FUNCTION "PALLET IMP.LAT. TRANSITO" : VOID
TITLE =
VERSION : 0.1
//KNOW_HOW_PROTECT

VAR_TEMP
  Error_block_move : INT ;
END_VAR
BEGIN
NETWORK
TITLE =Spostamento dati per pallet in transito tra impil. e ribaltat.
//- "Container Flag"
//- "Id TAG"
//- "FlagRibaltamento"
//- "Container_Id"
//- "Date LCB"
//- "Part Number"
//- "Quantity"
//- "Line Id"
//- "CIM"
//- "Colata Id"
//- "Material Of Test Flag"
//- "Lotto Id"
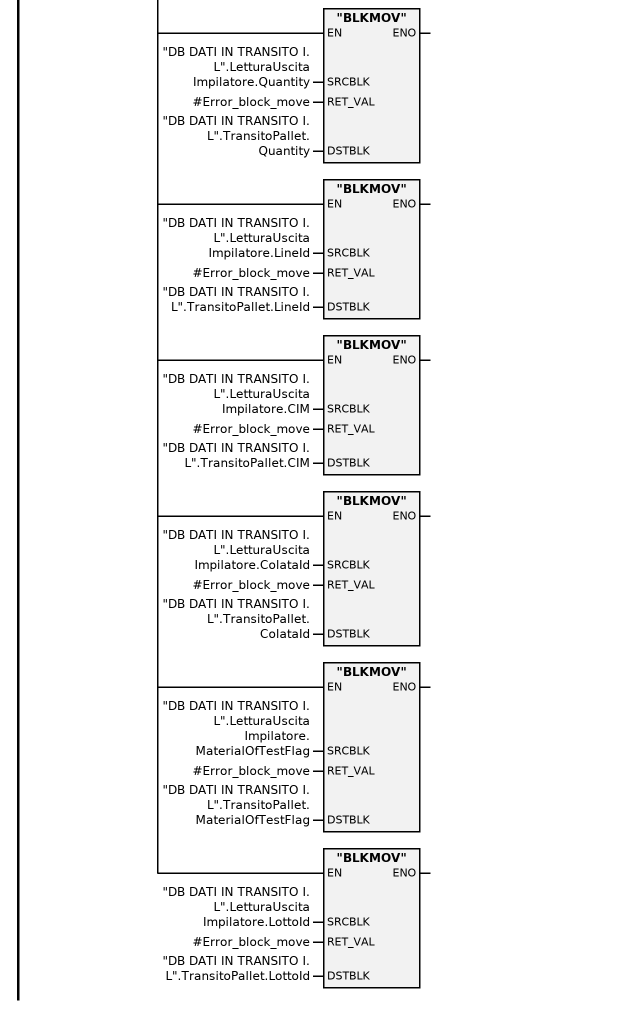
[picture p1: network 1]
      U     "DB SCAMBIO DATI PIANELLI".Trasl_ped_da_I_L_a_ribal;
      =     L      2.0;
      U     L      2.0;
      SPBNB _001;
      CALL "BLKMOV" (
           SRCBLK                   := "DB DATI IN TRANSITO I. L".LetturaUscitaImpilatore.ContainerFlag,
           RET_VAL                  := #Error_block_move,
           DSTBLK                   := "DB DATI IN TRANSITO I. L".TransitoPallet.ContainerFlag);
_001: NOP   0;
      U     L      2.0;
      SPBNB _002;
      CALL "BLKMOV" (
           SRCBLK                   := "DB DATI IN TRANSITO I. L".LetturaUscitaImpilatore.ID_TAG,
           RET_VAL                  := #Error_block_move,
           DSTBLK                   := "DB DATI IN TRANSITO I. L".TransitoPallet.ID_TAG);
_002: NOP   0;
      U     L      2.0;
      SPBNB _003;
      CALL "BLKMOV" (
           SRCBLK                   := "DB DATI IN TRANSITO I. L".LetturaUscitaImpilatore.FlagRibaltamento,
           RET_VAL                  := #Error_block_move,
           DSTBLK                   := "DB DATI IN TRANSITO I. L".TransitoPallet.FlagRibaltamento);
_003: NOP   0;
      U     L      2.0;
      SPBNB _004;
      CALL "BLKMOV" (
           SRCBLK                   := "DB DATI IN TRANSITO I. L".LetturaUscitaImpilatore.Container_Id,
           RET_VAL                  := #Error_block_move,
           DSTBLK                   := "DB DATI IN TRANSITO I. L".TransitoPallet.Container_Id);
_004: NOP   0;
      U     L      2.0;
      SPBNB _005;
      CALL "BLKMOV" (
           SRCBLK                   := "DB DATI IN TRANSITO I. L".LetturaUscitaImpilatore.DateLCB,
           RET_VAL                  := #Error_block_move,
           DSTBLK                   := "DB DATI IN TRANSITO I. L".TransitoPallet.DateLCB);
_005: NOP   0;
      U     L      2.0;
      SPBNB _006;
      CALL "BLKMOV" (
           SRCBLK                   := "DB DATI IN TRANSITO I. L".LetturaUscitaImpilatore.PartNumber,
           RET_VAL                  := #Error_block_move,
           DSTBLK                   := "DB DATI IN TRANSITO I. L".TransitoPallet.PartNumber);
_006: NOP   0;
      U     L      2.0;
      SPBNB _007;
      CALL "BLKMOV" (
           SRCBLK                   := "DB DATI IN TRANSITO I. L".LetturaUscitaImpilatore.Quantity,
           RET_VAL                  := #Error_block_move,
           DSTBLK                   := "DB DATI IN TRANSITO I. L".TransitoPallet.Quantity);
_007: NOP   0;
      U     L      2.0;
      SPBNB _008;
      CALL "BLKMOV" (
           SRCBLK                   := "DB DATI IN TRANSITO I. L".LetturaUscitaImpilatore.LineId,
           RET_VAL                  := #Error_block_move,
           DSTBLK                   := "DB DATI IN TRANSITO I. L".TransitoPallet.LineId);
_008: NOP   0;
      U     L      2.0;
      SPBNB _009;
      CALL "BLKMOV" (
           SRCBLK                   := "DB DATI IN TRANSITO I. L".LetturaUscitaImpilatore.CIM,
           RET_VAL                  := #Error_block_move,
           DSTBLK                   := "DB DATI IN TRANSITO I. L".TransitoPallet.CIM);
_009: NOP   0;
      U     L      2.0;
      SPBNB _00a;
      CALL "BLKMOV" (
           SRCBLK                   := "DB DATI IN TRANSITO I. L".LetturaUscitaImpilatore.ColataId,
           RET_VAL                  := #Error_block_move,
           DSTBLK                   := "DB DATI IN TRANSITO I. L".TransitoPallet.ColataId);
_00a: NOP   0;
      U     L      2.0;
      SPBNB _00b;
      CALL "BLKMOV" (
           SRCBLK                   := "DB DATI IN TRANSITO I. L".LetturaUscitaImpilatore.MaterialOfTestFlag,
           RET_VAL                  := #Error_block_move,
           DSTBLK                   := "DB DATI IN TRANSITO I. L".TransitoPallet.MaterialOfTestFlag);
_00b: NOP   0;
      U     L      2.0;
      SPBNB _00c;
      CALL "BLKMOV" (
           SRCBLK                   := "DB DATI IN TRANSITO I. L".LetturaUscitaImpilatore.LottoId,
           RET_VAL                  := #Error_block_move,
           DSTBLK                   := "DB DATI IN TRANSITO I. L".TransitoPallet.LottoId);
_00c: NOP   0;
NETWORK
TITLE =
//m20000.0 = Tag corrispondente
//
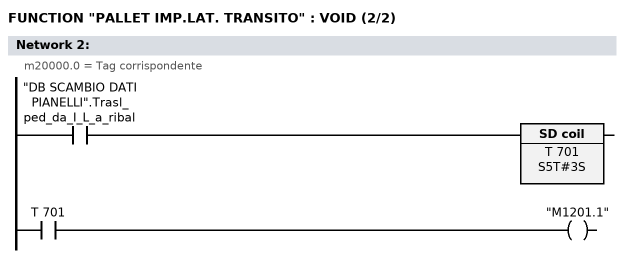
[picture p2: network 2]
      U     "DB SCAMBIO DATI PIANELLI".Trasl_ped_da_I_L_a_ribal;
      L     S5T#3S;
      SE    T    701;
      NOP   0;
      NOP   0;
      NOP   0;
      U     T    701;
      =     "M1201.1";
END_FUNCTION

